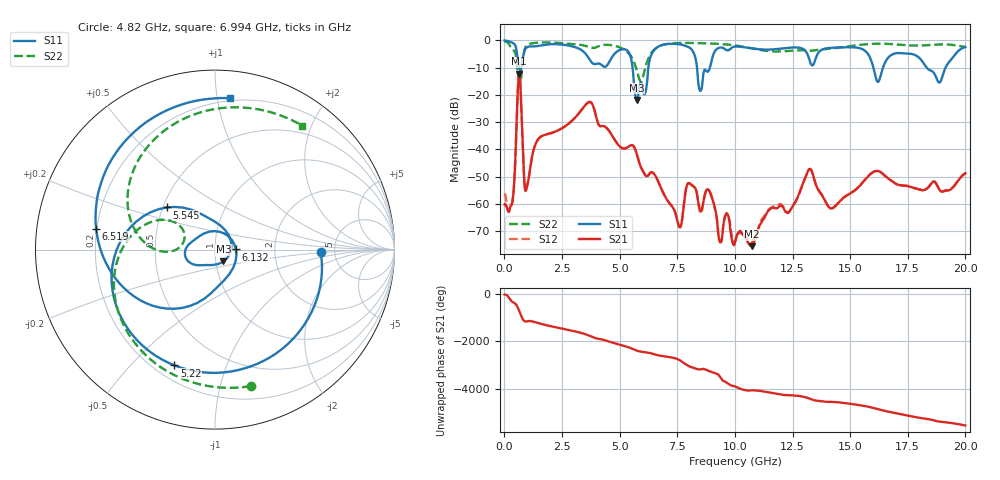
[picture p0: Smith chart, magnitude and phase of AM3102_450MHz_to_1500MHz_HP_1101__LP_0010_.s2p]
!Agilent Technologies,E8364B,MY43040894,A.07.50.67
!Agilent E8364B: A.07.50.67
!Date: Thursday, January 11, 2018 06:37:40
!Correction: S11(Full 2 Port(1,2))
!S21(Full 2 Port(1,2))
!S12(Full 2 Port(1,2))
!S22(Full 2 Port(1,2))
!S2P File: Measurements: S11, S21, S12, S22:
# Hz S  dB  R 50
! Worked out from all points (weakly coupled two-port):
!   1601 points, 10 MHz to 20 GHz, reference 50 ohm
!   highest |S21| = -12.29 dB at 647.2 MHz (marker M1); lowest = -75.4 dB at 10.73 GHz (marker M2)
!   lowest |S11| = -21.8 dB at 5.745 GHz (marker M3), VSWR 1.18, Z = 54.4 - j7.23 ohm
!   |S11| at or under -10 dB: 5.561 GHz to 6.245 GHz (684.7 MHz wide, 11.6 % of centre); 8.357 GHz to 8.916 GHz (559 MHz wide, 6.47 % of centre); 18.32 GHz to 19.14 GHz (818.3 MHz wide, 4.37 % of centre)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
!   |S22| runs from -15.4 to -0.3 dB; largest |S21 - S12| = 0.001
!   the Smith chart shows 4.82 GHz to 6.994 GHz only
!   S11 on the Smith chart (normalised r, x): 4.82 GHz: 3.86, -0.18; 5.22 GHz: 0.28, -0.67; 5.545 GHz: 0.52, +0.28; 6.132 GHz: 1.26, +0.00; 6.519 GHz: 0.20, +0.08; 6.994 GHz: 0.18, +1.09
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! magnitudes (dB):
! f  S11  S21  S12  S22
! 10 MHz  -0.1  -60.1  -56.1  -0.3
! 334.8 MHz  -0.8  -59.8  -59.5  -3.2
! 647.2 MHz  -10.3  -12.3  -12.3  -15.3
! 959.5 MHz  -2.7  -54.3  -54.2  -2.0
! 1.472 GHz  -2.1  -36.2  -36.2  -0.9
! 3.346 GHz  -3.6  -25.5  -25.5  -1.7
! 4.82 GHz  -4.6  -36.9  -36.9  -2.1
! 5.22 GHz  -3.3  -39.6  -39.6  -3.5
! 5.545 GHz  -8.9  -38.4  -38.4  -6.6
! 5.745 GHz  -21.8  -41.7  -41.7  -11.1
! 6.132 GHz  -18.7  -49.6  -49.6  -9.4
! 6.519 GHz  -3.4  -49.2  -49.2  -3.3
! 6.682 GHz  -2.3  -51.9  -51.9  -2.4
! 6.994 GHz  -1.4  -57.5  -57.6  -1.5
! 8.493 GHz  -18.5  -62.4  -62.9  -1.1
! 10.01 GHz  -2.3  -73.7  -73.9  -1.9
! 10.73 GHz  -2.9  -75.4  -74.2  -3.0
! 13.34 GHz  -9.1  -48.1  -48.1  -3.8
! 14.18 GHz  -2.8  -61.7  -61.5  -3.0
! 16.68 GHz  -6.1  -50.7  -50.8  -1.3
! 18.86 GHz  -15.5  -54.6  -54.6  -1.5
! 20 GHz  -2.5  -48.7  -48.8  -2.4
